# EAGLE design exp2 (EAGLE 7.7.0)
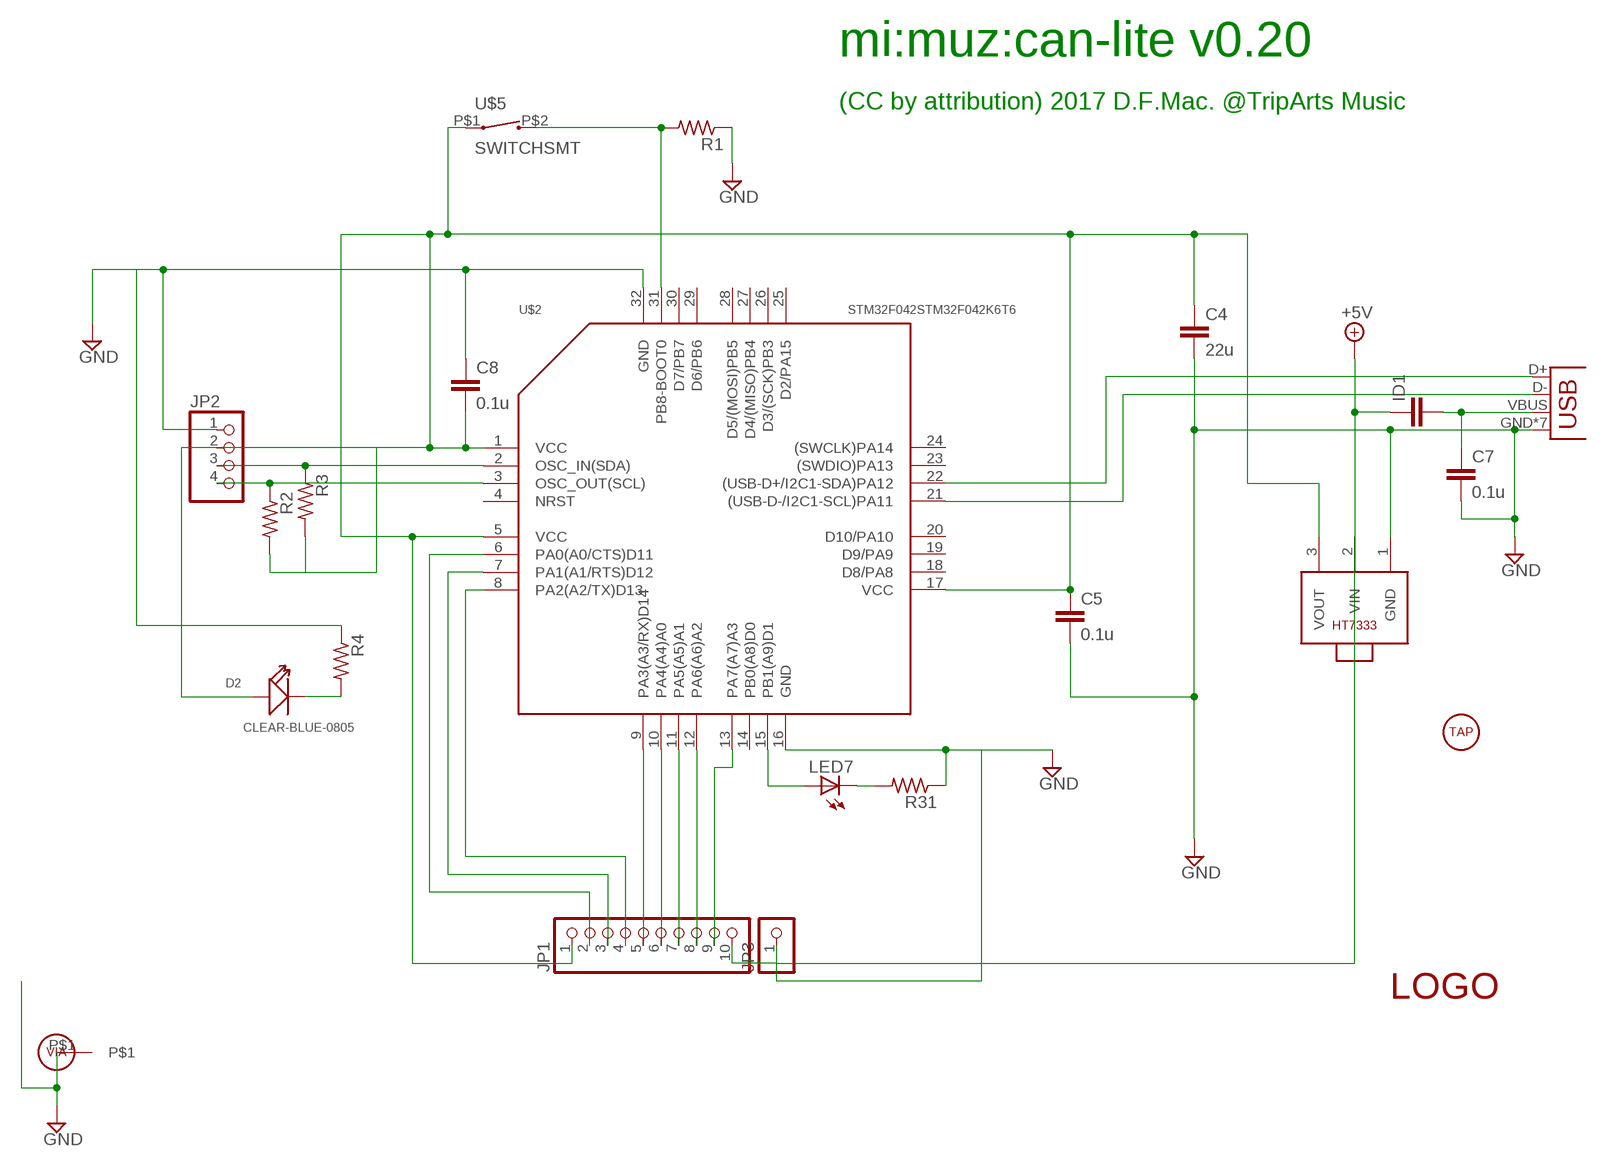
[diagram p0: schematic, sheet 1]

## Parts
C4  22u  C-EUC0805  [C0805]
C5  0.1u  C-EUC0603  [C0603]
C7  0.1u  C-EUC0603  [C0603]
C8  0.1u  C-EUC0603  [C0603]
D2  CLEAR-BLUE-0805  SMD-LED-CLEAR-BLUE(0805)  [LED-0805]
ID1  C-EUC0805  [C0805]
JP1  PINHD-1X10  [1X10]
JP2  PINHD-1X4  [1X04]
JP3  PINHD-1X1NORMAL  [1X01S]
JP4  USB-MICROB  [USB-MICROB]
LED7  LED3MM  [LED3MM]
R1  R-US_R0603  [R0603]
R2  R-US_R0603  [R0603]
R3  R-US_R0603  [R0603]
R4  R-US_R0603  [R0603]
R31  R-US_R0603  [R0603]
U$1  LOGOSMALL  [LOGO-SMALL]
U$2  STM32F042STM32F042K6T6  [TQFP32]
U$3  TAPHOLE  [TAPHOLE-3MM]
U$4  VIA  [VIA]
U$5  SWITCHSMT  [SWITCH-SMT-2*4*3]
U$14  HT7333  [SOT89]

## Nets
3.3V: C4.1 C5.1 C8.2 D2.+ JP1.1 JP2.2 R2.2 R3.2 U$2.1(VCC) U$2.5(VCC) U$2.17(VCC) U$5.P$1 U$14.3(VOUT)
+5V: ID1.1 JP1.10 U$14.2(VIN)
D+: JP4.D+ U$2.22((USB-D+/I2C1-SDA)PA12)
D-: JP4.D- U$2.21((USB-D-/I2C1-SCL)PA11)
GND [power]: C4.2 C5.2 C7.2 C8.1 JP2.1 JP3.1 JP4.GND JP4.MT1(GND) JP4.MT3(GND) JP4.P$2(GND) JP4.P$4(GND) JP4.P$5(GND) JP4.P$6(GND) R1.1 R4.1 R31.1 U$2.16(GND) U$2.32(GND) U$4.P$1 U$14.1(GND)
N$1: LED7.A U$2.15(PB1(A9)D1)
N$2: LED7.K(C) R31.2
N$3: JP1.2 U$2.6(PA0(A0/CTS)D11)
N$4: JP1.3 U$2.7(PA1(A1/RTS)D12)
N$5: JP1.4 U$2.8(PA2(A2/TX)D13)
N$6: JP1.5 U$2.9(PA3(A3/RX)D14)
N$7: JP1.6 U$2.10(PA4(A4)A0)
N$8: JP1.7 U$2.11(PA5(A5)A1)
N$9: JP1.8 U$2.12(PA6(A6)A2)
N$10: JP1.9 U$2.13(PA7(A7)A3)
N$11: JP2.3 R3.1 U$2.2(OSC_IN(SDA))
N$12: JP2.4 R2.1 U$2.3(OSC_OUT(SCL))
N$13: D2.- R4.2
N$30: R1.2 U$2.31(PB8-BOOT0) U$5.P$2
VBUS: C7.1 ID1.2 JP4.VBUS
Unconnected: U$2.4(NRST) U$2.14(PB0(A8)D0) U$2.18(D8/PA8) U$2.19(D9/PA9) U$2.20(D10/PA10) U$2.23((SWDIO)PA13) U$2.24((SWCLK)PA14) U$2.25(D2/PA15) U$2.26(D3/(SCK)PB3) U$2.27(D4/(MISO)PB4) U$2.28(D5/(MOSI)PB5) U$2.29(D6/PB6) U$2.30(D7/PB7)

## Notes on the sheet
- mi:muz:can-lite v0.20
- (CC by attribution) 2017 D.F.Mac. @TripArts Music

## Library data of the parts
C4 C5 C7 C8 ID1 = 0my:C-EU: CAPACITOR, European symbol
D2 = Seeed-OPL-Diode:SMD-LED-CLEAR-BLUE(0805): 304090061; MPN: EL-17-215/BHC-AN1P2/3T
JP1 = 0my:PINHD-1X10: PIN HEADER
JP2 = 0my:PINHD-1X4: PIN HEADER
JP3 = 0my:PINHD-1X1: PIN HEADER
JP4 = 0my:USB: USB Connectors USB-B-PTH is fully proven SKU : PRT-00139/CONN-08278 USB-miniB is fully proven SKU : PRT-00587 USB-A-PCB is untested. USB-A-H is throughly reviewed, but untested. Spark Fun Electronics SKU : PRT-00437 USB-B-SMT is throughly reviewed, but untested. Needs silkscreen touching up.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; PROD_ID: CONN-09505
LED7 = led:LED: LED
R1-R4 R31 = 0my:R-US_: RESISTOR, American symbol
U$1 = 0my:LOGO
U$2 = 1my:STM32F042
U$3 = 0my:TAPHOLE
U$4 = 0my:VIA
U$5 = 1my:SWITCH
U$14 = 0my:HT7333

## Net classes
0 default: width 0.406 mm, clearance 0.254 mm
1 power: width 0.533 mm, clearance 0.254 mm
2 D+: width 0.305 mm, clearance 0.203 mm
3 D-: width 0.305 mm, clearance 0.203 mm
4 VBUS: width 0.406 mm, clearance 0.203 mm

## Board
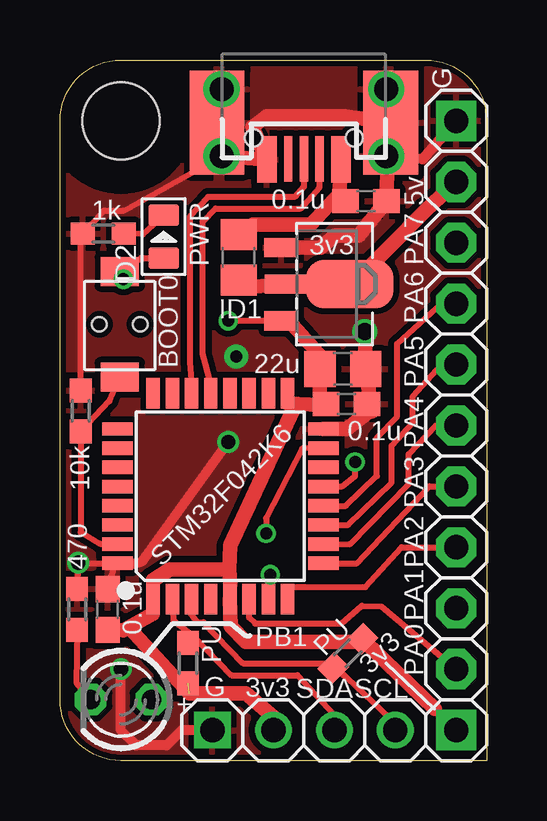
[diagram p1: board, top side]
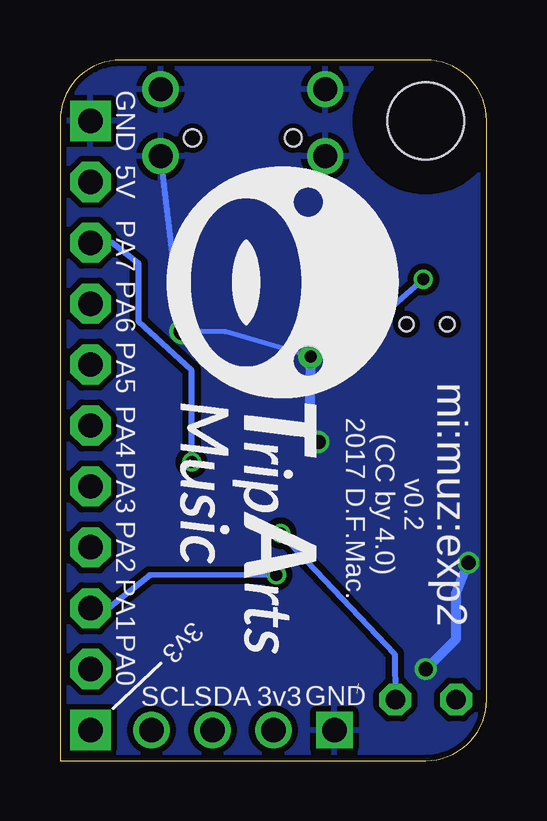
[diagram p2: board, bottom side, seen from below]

Size 17.78 x 29.21 mm. Coordinates in mm from the lower left corner, seen from the top.
Outline: 17.78,0 2.54,0 arc-90 0,2.54 0,26.67 arc-90 2.54,29.21 15.24,29.21 arc-90 17.78,26.67 17.78,0
Copper layers (1*16): Top 0.035mm / dielectric 1.5mm / Bottom 0.035mm
Design rules "Elecrow_2-layer_eagle_rule": minimum track width 6mil, minimum drill 12mil, track to track 6mil, track to pad 6mil, pad to pad 6mil, via to via 6mil, smd to smd 0mil, copper to edge 10mil, drill to drill 10mil, minimum pad ring 10mil, minimum via ring 6mil, stop-mask expansion 2mil, vias tented up to drill 100mil, thermal gap 10mil

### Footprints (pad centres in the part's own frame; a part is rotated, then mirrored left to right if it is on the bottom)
C0805 = smd 1.3 x 1.5: 1 -0.95,0; 2 0.95,0
C0603 = smd 1.1 x 1: 1 -0.85,0; 2 0.85,0
LED-0805 = smd 0.889 x 1.27: + -0.889,0; - 0.889,0
1X10 = drill 1.016 pad 1.676 square: 1 -11.43,0 | drill 1.016 pad 1.676 octagon: 2 -8.89,0; 3 -6.35,0; 4 -3.81,0; 5 -1.27,0; 6 1.27,0; 7 3.81,0; 8 6.35,0; 9 8.89,0; 10 11.43,0
1X04 = drill 1.016 square: 1 -3.81,0 | drill 1.016: 2 -1.27,0; 3 1.27,0; 4 3.81,0
1X01S = drill 1.016 pad 1.676 square: 1 0,0
USB-MICROB = smd 0.35 x 1.9: D+ 0,2.904; D- -0.65,2.904; ID 0.65,2.904 | smd 0.813 x 1.93: GND 1.541,2.929; VBUS -1.541,2.929 | smd 2.286 x 4.318: MT1 3.62,1.397; MT3 -3.619,1.397 | drill 1: P$2 -3.429,2.794; P$4 -3.429,0; P$5 3.429,2.794; P$6 3.429,0 | hole 0.7: -2.095,2.032; 2.095,2.032
LED3MM = drill 0.813 octagon: A -1.27,0; K 1.27,0
R0603 = smd 1 x 0.9: 1 -0.85,0; 2 0.85,0
TQFP32 = smd 1.27 x 0.559: 1 -4.293,2.8; 2 -4.293,2; 3 -4.293,1.2; 4 -4.293,0.4; 5 -4.293,-0.4; 6 -4.293,-1.2; 7 -4.293,-2; 8 -4.293,-2.8; 17 4.293,-2.8; 18 4.293,-2; 19 4.293,-1.2; 20 4.293,-0.4; 21 4.293,0.4; 22 4.293,1.2; 23 4.293,2; 24 4.293,2.8 | smd 0.559 x 1.27: 9 -2.8,-4.293; 10 -2,-4.293; 11 -1.2,-4.293; 12 -0.4,-4.293; 13 0.4,-4.293; 14 1.2,-4.293; 15 2,-4.293; 16 2.8,-4.293; 25 2.8,4.293; 26 2,4.293; 27 1.2,4.293; 28 0.4,4.293; 29 -0.4,4.293; 30 -1.2,4.293; 31 -2,4.293; 32 -2.8,4.293
TAPHOLE-3MM = hole 3.2: 0,0
VIA = drill 0.5 pad 0.813: P$1 0,0
SWITCH-SMT-2*4*3 = smd 1.2 x 1.6: P$1 2.2,0; P$2 -2.2,0 | hole 0.6: 0,-0.85; 0,0.85
SOT89 = smd 0.8 x 1.4: 1 -1.524,-1.905; 3 1.524,-1.905 | smd 0.8 x 1.9: 2 0,-1.651 | smd 2.032 x 3.65: 4 0,0.94

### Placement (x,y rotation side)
C4  11.79,16.33 0 top
C5  11.94,14.86 0 top
C7  12.75,23.32 0 top
C8  1.98,6.3 270 top
D2  4.32,21.84 90 top
ID1  7.44,20.98 90 top
JP1  16.51,12.7 90 top
JP2  10.16,1.27 0 top
JP3  16.51,26.67 0 top
JP4  10.16,27.99 180 top
LED7  2.54,2.54 180 top
R1  0.86,14.58 270 top
R2  11.99,4.47 45 top
R3  5.33,4.06 270 top
R4  1.8,21.97 0 top
R31  0.71,6.3 270 top
U$1  13.34,24.77 270 bottom
U$2  6.68,11.02 90 top
U$3  2.54,26.67 0 top
U$4  7.34,16.84 0 top
U$5  2.49,18.19 90 top
U$14  11.13,19.86 270 top

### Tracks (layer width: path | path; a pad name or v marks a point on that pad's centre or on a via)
3.3V  (via drill 0.5)  (1 unrouted)
  Top 0.254: v2.64,20.07 U$5.P$1 3.38,20.95 D2.+ | v7.01,18.34 U$14.3 | R2.2 14.58,3.15
  Top 0.406: U$2.17 9.5,14.88 10.16,14.86 9.73,14.63 | 3.86,7.52 U$2.1 3.86,6.12 | 7.09,7.32 U$2.5 | JP1.1 15.62,2.16
  Top 0.61: U$14.3 9.7,18.16 10.95,16.76 C4.1 10.82,14.91 C5.1 10.87,14.83 9.5,14.88 | 9.73,14.63 7.09,8.97 7.06,7.98 | 7.06,7.98 4.57,7.98 3.86,7.52 | 7.06,7.98 7.09,7.32 | 15.62,2.16 14.58,3.15 12.7,4.95 7.75,4.95 7.11,5.59 U$2.5 | R2.2 14.13,3.58 | C8.2 2.64,5.44 2.87,5.56 | 2.87,5.56 3.86,6.12 | JP2.2 8.89,1.83 7.75,2.79 5.38,2.79 2.87,5.56
  Bottom 0.254: v2.64,20.07 4.6,18.34 v7.01,18.34
+5V
  Top 0.61: ID1.1 7.57,19.71 U$14.2 12.19,19.86 15.21,22.94 JP1.10
D+
  Top 0.254: JP4.D+ 10.16,23.93 9.78,23.5 6.17,23.5 5.41,22.68 5.41,16.61 5.49,15.6 U$2.22
D-
  Top 0.254: U$2.21 6.27,15.72 5.94,16.94 5.94,22.48 6.48,23.01 10.03,23.01 10.82,23.9 10.82,24.38 JP4.D-
GND  (via drill 0.6, 0.7)
  Top 0.254: R31.1 0.79,8.23 | 0.79,8.23 2.36,8.23 | C8.1 2.26,8.05 2.39,8.15 | 2.36,8.23 2.39,8.15 | 2.39,8.15 U$2.32 | R1.1 0.86,21.84 1.33,22.37 | 1.33,22.37 1.83,22.94 2.67,22.94 JP4.P$5 | 2.36,8.23 2.97,8.23 | v0.76,8.26 0.79,8.23 | R4.1 1.33,22.37
  Top 0.406: JP4.P$2 15.11,25.07 JP3.1 | 2.97,8.23 3.17,8.23 3.43,8.31 v7.01,13.28 | JP2.1 5.08,1.27 4.45,0.64 3.17,0.64 2.54,1.27 v2.54,3.81
  Top 0.61: U$14.1 10.87,21.39 11.46,21.89 12.45,21.89 C7.2 13.64,24.46 13.64,24.74 JP4.P$2 JP4.MT3 | JP4.MT3 JP4.P$4 | JP4.P$6 JP4.MT1 JP4.P$5 JP4.GND 8,26.42 8.61,26.87 11.86,26.87 JP4.MT3 | U$2.16 11.94,13.82 12.9,14.58 C5.2 12.98,14.55 C4.2 v12.7,17.88
  Bottom 0.203: U$4.P$1 10.9,17.88 v12.7,17.88
  Bottom 0.254: v12.7,17.88 JP4.P$2
  Bottom 0.406: v7.01,13.28 7.37,13.82 U$4.P$1 | v2.54,3.81 1.27,5.08 1.27,6.99 v0.76,8.26
  pour Top: -0.64,29.21 18.41,29.21 18.41,0 -0.64,0
  pour Bottom: 0,29.84 17.78,29.84 17.78,-0.64 0,-0.64
N$1  (via drill 0.5)
  Top 0.254: U$2.15 10.08,13.01 8.59,10.11 v8.59,9.47
  Bottom 0.254: v8.59,9.47 3.83,4.45 LED7.A
N$2
  Top 0.254: R31.2 0.69,3.25 LED7.K
N$3
  Top 0.254: U$2.6 7.87,5.97 8.13,5.71 11.73,5.71 12.57,6.45 13.39,6.43 JP1.2
N$4  (via drill 0.5)
  Top 0.254: U$2.7 8.69,7.44 v8.76,7.75
  Bottom 0.254: v8.76,7.75 14.05,7.72 15.77,6.35 JP1.3
N$5
  Top 0.254: U$2.8 9.47,7.06 9.65,7.24 12.72,7.24 14.22,8.89 JP1.4
N$6
  Top 0.254: U$2.9 12.37,8.23 15.39,11.43 JP1.5
N$7
  Top 0.254: U$2.10 12.06,9.02 14.53,11.53 14.53,12.78 15.65,13.97 JP1.6
N$8
  Top 0.254: U$2.11 12.01,9.83 13.82,11.58 13.82,13.13 14.71,14.1 14.71,15.19 15.88,16.51 JP1.7
N$9
  Top 0.254: U$2.12 11.91,10.62 13.21,11.86 13.21,13.46 14.05,14.35 14.05,17.37 15.93,19.07 JP1.8
N$10  (via drill 0.5)
  Top 0.254: U$2.13 11.76,11.43 12.29,11.86 v12.29,12.45
  Bottom 0.254: v12.29,12.45 12.29,16.28 14.5,18.31 14.5,20.73 15.65,21.61 JP1.9
N$11
  Top 0.254: U$2.2 4.72,5.84 5.6,5.17 | 5.6,5.17 7.14,3.56 9.91,3.56 11.43,1.91 JP2.3 | R3.1 5.6,5.17
N$12
  Top 0.254: U$2.3 5.46,6.1 5.71,5.77 5.97,5.77 7.62,4.06 11.3,4.06 11.96,3.45 | 11.96,3.45 13.72,1.78 JP2.4 | R2.1 11.96,3.45
N$13
  Top 0.254: D2.- 3.45,21.95 R4.2
N$30
  Top 0.254: U$5.P$2 2.06,14.99 R1.2 0.86,9.53 1.68,9.04 U$2.31
VBUS
  Top 0.61: JP4.VBUS 11.66,23.72 C7.1 11.68,23.67 10.44,22.35 8.03,22.35 ID1.2

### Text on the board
_tNames: G | 5v | 1k | 0.1u | PWR | 3v3 | PA7 | ID1 | PA6 | BOOT0 | 22u | PA5 | 0.1u | PA4 | 10k | PA3 | STM32F042K6 | 470 | PA2 | PA1 | 0.1u | PU | PB1 | PU | 3v3 | PA0 | G | 3v3 | SDA | SCL | +
_bNames: GND | 5V | PA7 | PA6 | PA5 | PA4 | mi:muz:exp2 | v0.2 / (CC by 4.0) / 2017 D.F.Mac. | PA3 | PA2 | PA1 | 3v3 | PA0 | GND | 3v3 | SDA | SCL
